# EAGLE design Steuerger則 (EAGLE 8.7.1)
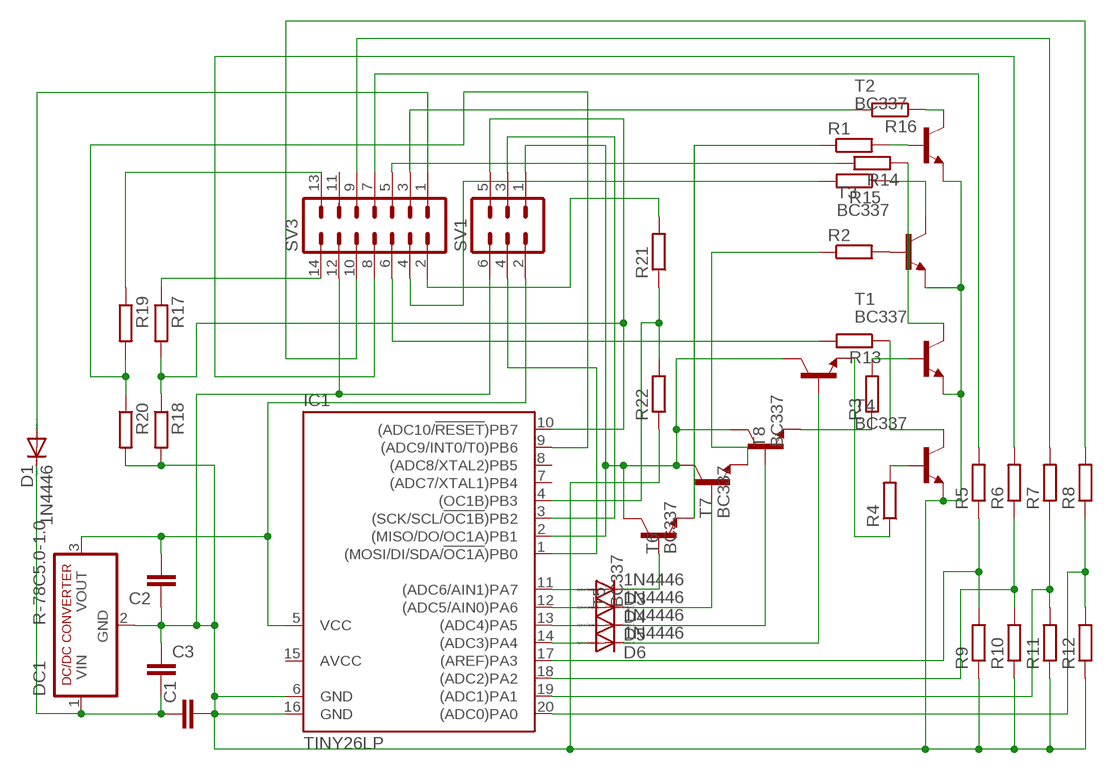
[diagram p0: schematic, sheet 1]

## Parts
C1  C5/3  [C5B3]
C2  C5/3  [C5B3]
C3  C5/3  [C5B3]
D1  1N4446  [DO35-10]
D3  1N4446  [DO35-10]
D4  1N4446  [DO35-10]
D5  1N4446  [DO35-10]
D6  1N4446  [DO35-10]
DC1  R-78C5.0-1.0  [SIP3]
IC1  TINY26LP  [DIL20]
R1  R-EU_0204/5  [0204/5]
R2  R-EU_0204/5  [0204/5]
R3  R-EU_0204/5  [0204/5]
R4  R-EU_0204/5  [0204/5]
R5  R-EU_0204/5  [0204/5]
R6  R-EU_0204/5  [0204/5]
R7  R-EU_0204/5  [0204/5]
R8  R-EU_0204/5  [0204/5]
R9  R-EU_0204/5  [0204/5]
R10  R-EU_0204/5  [0204/5]
R11  R-EU_0204/5  [0204/5]
R12  R-EU_0204/5  [0204/5]
R13  R-EU_0204/5  [0204/5]
R14  R-EU_0204/5  [0204/5]
R15  R-EU_0204/5  [0204/5]
R16  R-EU_0204/5  [0204/5]
R17  R-EU_0204/5  [0204/5]
R18  R-EU_0204/5  [0204/5]
R19  R-EU_0204/5  [0204/5]
R20  R-EU_0204/5  [0204/5]
R21  R-EU_0204/5  [0204/5]
R22  R-EU_0204/5  [0204/5]
SV1  ML6L  [ML6L]
SV3  ML14L  [ML14L]
T1  BC337  [TO92]
T2  BC337  [TO92]
T3  BC337  [TO92]
T4  BC337  [TO92]
T5  BC337  [TO92]
T6  BC337  [TO92]
T7  BC337  [TO92]
T8  BC337  [TO92]

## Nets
N$1: D1.A SV3.1
N$2: C2.2 DC1.3(VOUT) IC1.5(VCC) SV1.2
N$3: R17.1 SV3.14
N$4: IC1.3((SCK/SCL/!OC1B!)PB2) SV1.3
N$5: R19.1 SV3.13
N$6: IC1.1((MOSI/DI/SDA/!OC1A!)PB0) SV1.4
N$8: C1.2 C2.1 C3.1 DC1.2(GND) IC1.6(GND) IC1.16(GND) R9.1 R10.1 R11.1 R12.1 R18.2 R20.2 R22.1 SV1.6 SV3.12 T1.1(E) T2.1(E) T3.1(E) T4.1(E)
N$9: IC1.17((AREF)PA3) R5.1 R9.2
N$10: IC1.18((ADC2)PA2) R6.1 R10.2
N$11: IC1.19((ADC1)PA1) R7.1 R11.2
N$12: IC1.20((ADC0)PA0) R8.1 R12.2
N$14: D3.A IC1.11((ADC6/AIN1)PA7)
N$15: D4.A IC1.12((ADC5/AIN0)PA6)
N$16: D5.A IC1.13((ADC4)PA5)
N$17: D3.C T5.2(B)
N$18: D4.C T6.2(B)
N$19: D6.A IC1.14((ADC3)PA4)
N$20: R1.2 T2.2(B)
N$21: R2.2 T3.2(B)
N$22: R3.2 T1.2(B)
N$23: R4.2 T4.2(B)
N$24: D5.C T7.2(B)
N$25: D6.C T8.2(B)
N$26: R1.1 T5.1(E)
N$27: R2.1 T6.1(E)
N$28: R16.2 SV3.3
N$29: R15.2 SV3.4
N$30: R14.2 SV3.5
N$31: R13.2 SV3.6
N$32: R16.1 T2.3(C)
N$33: R13.1 T4.3(C)
N$34: R5.2 SV3.7
N$35: R6.2 SV3.8
N$36: R7.2 SV3.9
N$37: R8.2 SV3.10
N$38: R14.1 T1.3(C)
N$39: R15.1 T3.3(C)
N$40: R3.1 T7.1(E)
N$41: R4.1 T8.1(E)
N$42: IC1.9((ADC9/INT0/T0)PB6) R19.2 R20.1
N$43: C1.1 C3.2 D1.C DC1.1(VIN)
N$44: IC1.2((MISO/DO/OC1A)PB1) SV1.1 T5.3(C) T6.3(C) T7.3(C) T8.3(C)
N$45: IC1.10((ADC10/!RESET!)PB7) R17.2 R18.1 SV1.5
N$46: IC1.4((OC1B)PB3) R21.1 R22.2
N$47: R21.2 SV3.2
Unconnected: IC1.7((ADC7/XTAL1)PB4) IC1.8((ADC8/XTAL2)PB5) SV3.11

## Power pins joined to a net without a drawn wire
AVCC: IC1.15(AVCC)

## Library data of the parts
C1-C3 = capacitor-wima:C: CAPACITOR
D1 D3-D6 = diode:1N4446: DIODE
DC1 = dc-dc-converter:R-78C*-1.0: INNOLINE DC/DC-Converter 1.0 AMP SIP3 Single Output Source: Data sheet
IC1 = atmel:TINY26*: 8-bit AVR Microcontroller with 2K Bytes Flash Source: http://www.atmel.com .. doc1477.pdf; MPN: ATTINY26L-8PU; OC_FARNELL: 9171657; OC_NEWARK: 01M6920
R1-R4 R21 R22 = resistor:R-EU_: RESISTOR, European symbol
R5-R20 = rcl:R-EU_: RESISTOR, European symbol; SPICEPREFIX: R
SV1 = con-ml:ML6L: HARTING; OC_FARNELL: unknown; OC_NEWARK: unknown
SV3 = con-ml:ML14L: HARTING; OC_FARNELL: unknown; OC_NEWARK: unknown
T1-T8 = transistor:BC337: NPN TRANSISTOR

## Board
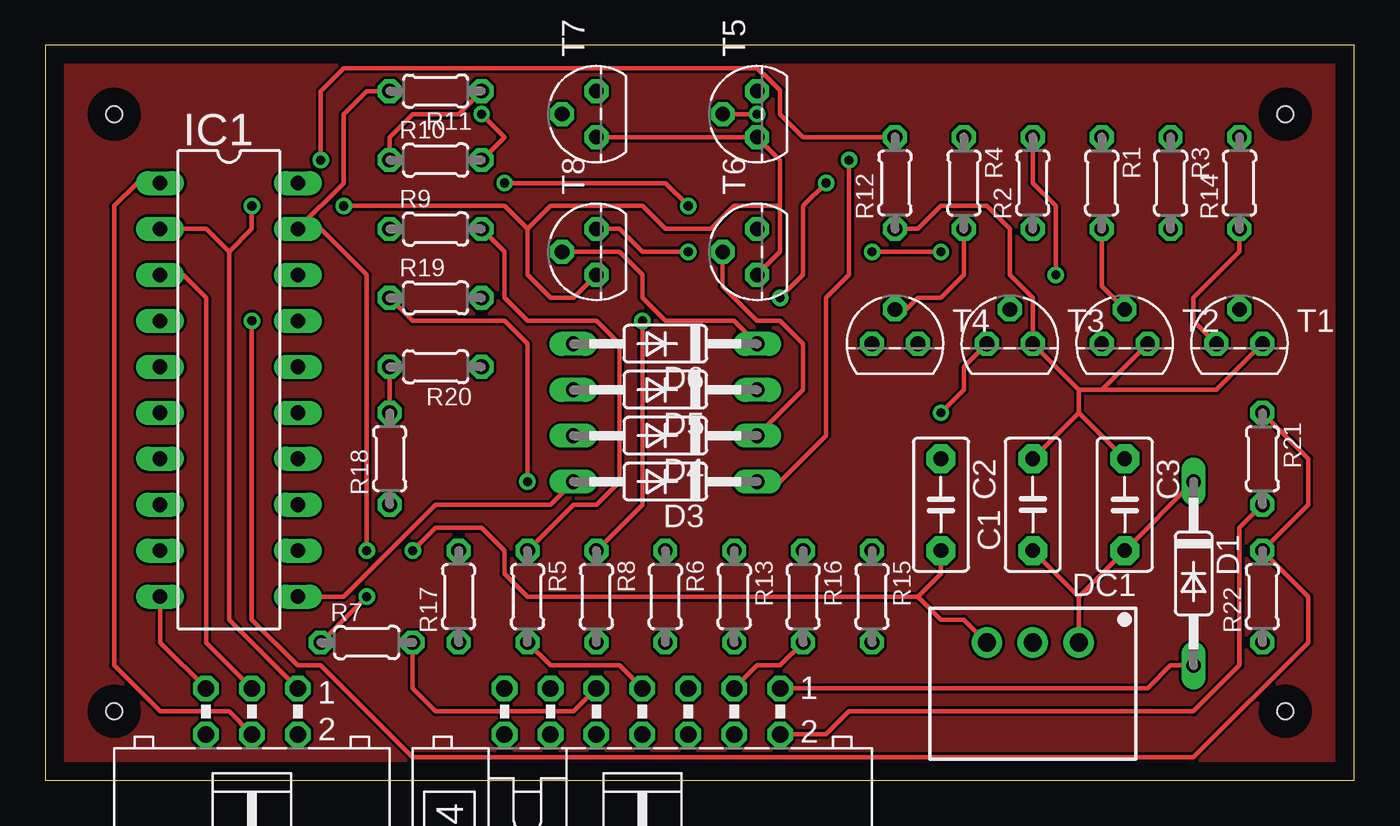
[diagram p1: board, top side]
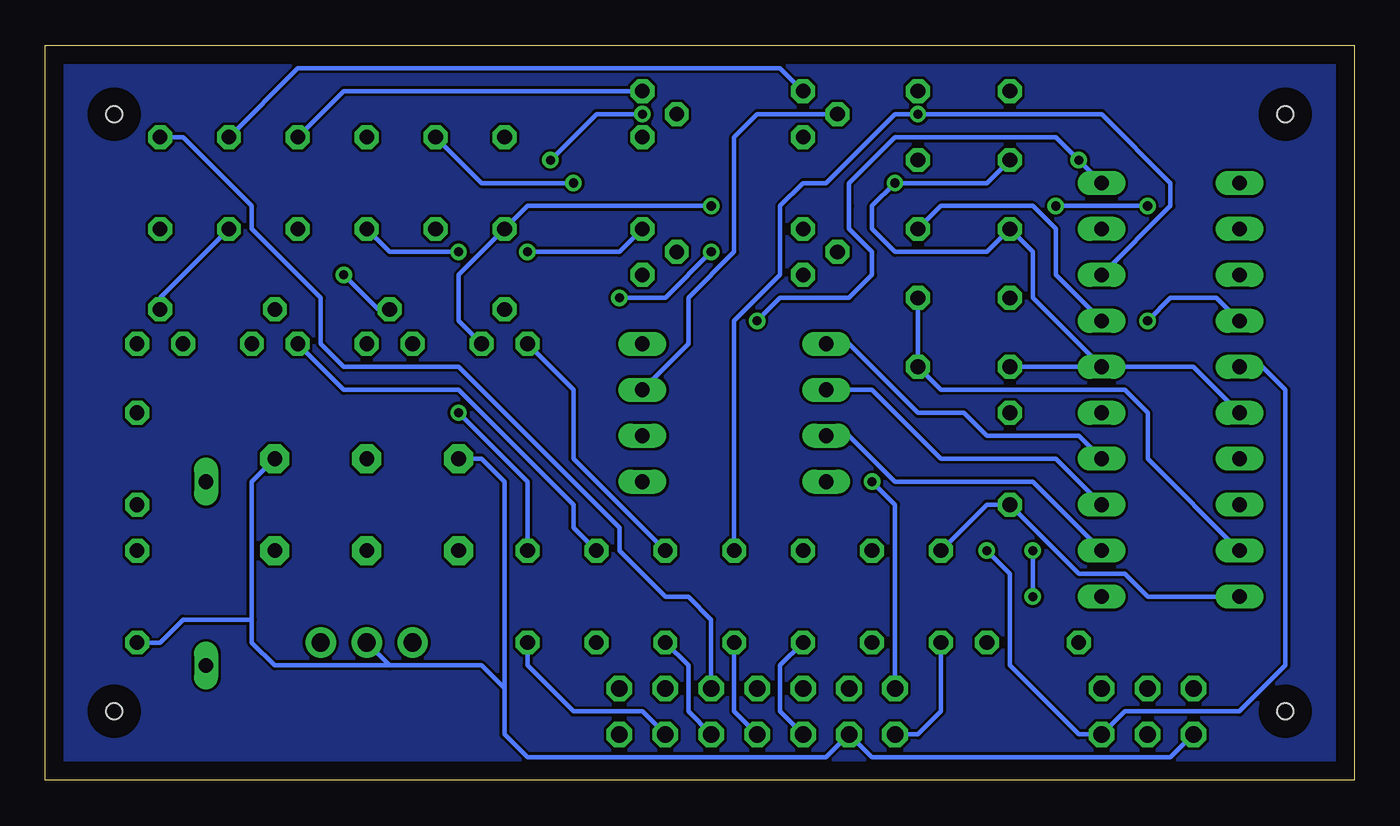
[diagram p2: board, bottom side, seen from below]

Size 72.39 x 40.64 mm. Coordinates in mm from the lower left corner, seen from the top.
Outline: 0,0 72.39,0 72.39,40.64 0,40.63 0,0
Copper layers (1*16): Top 0.035mm / dielectric 1.5mm / Bottom 0.035mm
Design rules "default": minimum track width 6mil, minimum drill 0.35mm, track to track 6mil, track to pad 6mil, pad to pad 6mil, via to via 6mil, smd to smd 6mil, copper to edge 40mil, drill to drill 6mil, minimum pad ring 10mil, minimum via ring 8mil, stop-mask expansion 4mil, vias tented up to drill 0mil, thermal gap 10mil
Holes 0.9 mm at 3.81,3.81 3.81,36.83 68.58,36.83 68.58,3.81

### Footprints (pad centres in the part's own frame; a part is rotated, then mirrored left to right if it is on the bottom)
C5B3 = drill 0.813 pad 1.6 octagon: 1 -2.54,0; 2 2.54,0
DO35-10 = drill 0.813 long: A 5.08,0; C -5.08,0
SIP3 = drill 1 pad 1.676: 1 -2.54,0; 2 0,0; 3 2.54,0
DIL20 = drill 0.813 long: 1 -11.43,-3.81; 2 -8.89,-3.81; 3 -6.35,-3.81; 4 -3.81,-3.81; 5 -1.27,-3.81; 6 1.27,-3.81; 7 3.81,-3.81; 8 6.35,-3.81; 9 8.89,-3.81; 10 11.43,-3.81; 11 11.43,3.81; 12 8.89,3.81; 13 6.35,3.81; 14 3.81,3.81; 15 1.27,3.81; 16 -1.27,3.81; 17 -3.81,3.81; 18 -6.35,3.81; 19 -8.89,3.81; 20 -11.43,3.81
0204/5 = drill 0.813 octagon: 1 -2.54,0; 2 2.54,0
ML6L = drill 0.914 octagon: 1 -2.54,-1.27; 2 -2.54,1.27; 3 0,-1.27; 4 0,1.27; 5 2.54,-1.27; 6 2.54,1.27
ML14L = drill 0.914 octagon: 1 -7.62,-1.27; 2 -7.62,1.27; 3 -5.08,-1.27; 4 -5.08,1.27; 5 -2.54,-1.27; 6 -2.54,1.27; 7 0,-1.27; 8 0,1.27; 9 2.54,-1.27; 10 2.54,1.27; 11 5.08,-1.27; 12 5.08,1.27; 13 7.62,-1.27; 14 7.62,1.27
TO92 = drill 0.813 octagon: 1 1.27,0; 2 0,1.905; 3 -1.27,0

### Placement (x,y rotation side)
C1  54.61,15.24 90 top
C2  49.53,15.24 270 top
C3  59.69,15.24 270 top
D1  63.5,11.43 270 top
D3  34.29,16.51 180 top
D4  34.29,19.05 180 top
D5  34.29,21.59 180 top
D6  34.29,24.13 180 top
DC1  54.61,7.62 180 top
IC1  10.16,21.59 270 top
R1  58.42,33.02 270 top
R2  54.61,33.02 90 top
R3  62.23,33.02 270 top
R4  50.8,33.02 270 top
R5  26.67,10.16 270 top
R6  34.29,10.16 270 top
R7  17.78,7.62 0 top
R8  30.48,10.16 270 top
R9  21.59,30.48 0 top
R10  21.59,34.29 0 top
R11  21.59,38.1 180 top
R12  46.99,33.02 90 top
R13  38.1,10.16 270 top
R14  66.04,33.02 90 top
R15  45.72,10.16 270 top
R16  41.91,10.16 270 top
R17  22.86,10.16 90 top
R18  19.05,17.78 90 top
R19  21.59,26.67 0 top
R20  21.59,22.86 180 top
R21  67.31,17.78 270 top
R22  67.31,10.16 90 top
SV1  11.43,3.81 180 top
SV3  33.02,3.81 180 top
T1  66.04,24.13 0 top
T2  59.69,24.13 0 top
T3  53.34,24.13 0 top
T4  46.99,24.13 0 top
T5  39.37,36.83 90 top
T6  39.37,29.21 90 top
T7  30.48,36.83 90 top
T8  30.48,29.21 90 top

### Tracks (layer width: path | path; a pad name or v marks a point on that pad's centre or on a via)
BOTTOM
  pour Bottom: 0,40.64 72.39,40.64 72.39,0 0,0
N$1
  Top 0.254: SV3.1 60.96,5.08 62.23,6.35 D1.A
N$2  (via drill 0.5)
  Top 0.254: v20.32,12.7 21.59,13.97 24.13,13.97 25.4,12.7 25.4,11.43 26.67,10.16 48.26,10.16 | 48.26,10.16 49.53,11.43 C2.2 | 48.26,10.16 49.53,8.89 50.8,8.89 DC1.3
  Bottom 0.254: IC1.5 5.08,22.86 3.81,21.59 3.81,6.35 6.35,3.81 12.7,3.81 SV1.2 15.24,2.54 19.05,6.35 19.05,11.43 v20.32,12.7
N$3
  Bottom 0.254: R17.1 22.86,3.81 24.13,2.54 SV3.14
N$4
  Top 0.254: IC1.3 7.62,27.94 8.89,26.67 8.89,7.62 SV1.3
N$5  (via drill 0.5)
  Top 0.254: v26.67,16.51 26.67,24.13 25.4,25.4 20.32,25.4 R19.1
  Bottom 0.254: SV3.13 25.4,15.24 v26.67,16.51
N$6
  Top 0.254: IC1.1 5.08,33.02 3.81,31.75 3.81,6.35 6.35,3.81 10.16,3.81 SV1.4
N$8  (via drill 0.5)
  Top 0.254: R20.2 R18.2 | R10.1 19.05,35.56 20.32,36.83 22.86,36.83 R11.1 | v35.56,31.75 34.29,33.02 v25.4,33.02 | R12.1 48.26,30.48 49.53,31.75 52.07,31.75 53.34,30.48 53.34,27.94 54.61,26.67 T3.1 57.15,21.59 | 57.15,21.59 58.42,21.59 | 58.42,21.59 T2.1 | 58.42,21.59 64.77,21.59 T1.1 | 57.15,21.59 57.15,20.32 | 57.15,20.32 C1.2 | C3.1 57.15,20.32
  Bottom 0.254: SV1.6 10.16,1.27 26.67,1.27 SV3.12 29.21,1.27 45.72,1.27 46.99,2.54 46.99,5.08 | 46.99,5.08 46.99,16.51 48.26,17.78 C2.1 | 46.99,5.08 48.26,6.35 53.34,6.35 | 53.34,6.35 DC1.2 | 53.34,6.35 59.69,6.35 60.96,7.62 60.96,8.89 | 60.96,8.89 60.96,16.51 C3.1 | IC1.6 8.89,22.86 IC1.16 | IC1.16 R20.2 | IC1.16 17.78,26.67 17.78,29.21 R9.1 20.32,29.21 25.4,29.21 26.67,30.48 26.67,31.75 v25.4,33.02 20.32,33.02 R10.1 | T4.1 49.53,25.4 49.53,27.94 R12.1 45.72,31.75 v35.56,31.75 | R22.1 66.04,7.62 64.77,8.89 60.96,8.89
N$9
  Top 0.254: R5.1 29.21,15.24 30.48,15.24 31.75,16.51 31.75,24.13 30.48,25.4 26.67,25.4 25.4,26.67 25.4,29.21 R9.2
  Bottom 0.254: IC1.17 16.51,27.94 16.51,30.48 17.78,31.75 22.86,31.75 R9.2
N$10  (via drill 0.5)
  Top 0.254: R10.2 25.4,35.56 v24.13,36.83
  Bottom 0.254: IC1.18 10.16,31.75 10.16,33.02 13.97,36.83 v24.13,36.83 25.4,36.83 29.21,33.02 30.48,33.02 31.75,31.75 31.75,27.94 34.29,25.4 R6.1
N$11  (via drill 0.5)
  Top 0.254: R11.2 17.78,38.1 16.51,36.83 16.51,33.02 IC1.19 15.24,30.48 17.78,27.94 v17.78,12.7 | R7.1 v17.78,10.16
  Bottom 0.254: v17.78,10.16 v17.78,12.7
N$12  (via drill 0.5)
  Top 0.254: R8.1 33.02,15.24 v33.02,25.4 | R12.2 41.91,35.56 40.64,36.83 40.64,38.16 39.76,39.04 39.7,39.04 39.37,39.37 16.51,39.37 15.24,38.1 v15.24,34.29
  Bottom 0.254: v33.02,25.4 31.75,26.67 27.94,26.67 26.67,27.94 26.67,29.21 27.94,30.48 27.94,31.75 27.94,33.02 25.4,35.56 16.51,35.56 v15.24,34.29 IC1.20
N$14
  Top 0.254: IC1.11 16.51,10.16 21.59,15.24 27.94,15.24 D3.A
N$15
  Bottom 0.254: IC1.12 17.78,16.51 25.4,16.51 27.94,19.05 D4.A
N$16
  Bottom 0.254: IC1.13 16.51,17.78 22.86,17.78 26.67,21.59 D5.A
N$17  (via drill 0.5)
  Top 0.254: T5.2 v39.37,36.83 | v44.45,34.29 44.45,27.94 43.18,26.67 43.18,19.05 40.64,16.51 D3.C
  Bottom 0.254: v39.37,36.83 41.91,36.83 v44.45,34.29
N$18
  Top 0.254: T6.2 37.47,27.31 39.37,25.4 40.64,25.4 41.91,24.13 41.91,21.59 D4.C
N$19
  Bottom 0.254: IC1.14 15.24,19.05 20.32,19.05 21.59,20.32 24.13,20.32 27.94,24.13 D6.A
N$20
  Top 0.254: R1.2 58.42,27.31 T2.2
N$21  (via drill 0.5)
  Top 0.254: R2.2 54.61,33.02 55.88,31.75 v55.88,27.94
  Bottom 0.254: v55.88,27.94 53.98,26.04 T3.2
N$22
  Bottom 0.254: R3.2 66.04,26.67 T1.2
N$23
  Top 0.254: T4.2 47.62,26.04 48.26,26.67 49.53,26.67 50.8,27.94 R4.2
N$24
  Bottom 0.254: T7.2 33.02,36.83 34.29,35.56 34.29,29.21 36.83,26.67 36.83,24.13 D5.C
N$25
  Top 0.254: D6.C 38.1,25.4 34.29,25.4 33.02,26.67 33.02,27.94 31.75,29.21 T8.2
N$26
  Bottom 0.254: T5.1 55.88,38.1 R1.1
N$27  (via drill 0.5)
  Top 0.254: v49.53,29.21 v45.72,29.21
  Bottom 0.254: R2.1 53.34,29.21 v49.53,29.21 | v45.72,29.21 40.64,29.21 T6.1
N$28
  Top 0.254: R16.2 40.64,6.35 39.37,6.35 SV3.3
N$29
  Bottom 0.254: R15.2 45.72,6.35 43.18,3.81 39.37,3.81 SV3.4
N$30
  Bottom 0.254: SV3.5 35.56,8.89 36.83,10.16 38.1,10.16 40.64,12.7 40.64,13.97 49.53,22.86 55.88,22.86 57.15,24.13 57.15,26.67 60.96,30.48 60.96,31.75 64.77,35.56 R14.2
N$31
  Bottom 0.254: R13.2 36.83,6.35 36.83,3.81 SV3.6
N$32
  Bottom 0.254: R16.1 43.18,13.97 43.18,15.24 49.53,21.59 55.88,21.59 T2.3
N$33
  Bottom 0.254: T4.3 43.18,21.59 43.18,17.78 R13.1
N$34
  Top 0.254: R5.2 27.94,6.35 31.75,6.35 SV3.7
N$35
  Bottom 0.254: R6.2 34.29,3.81 SV3.8
N$36
  Top 0.254: SV3.9 29.21,3.81 21.59,3.81 20.32,5.08 R7.2
N$37
  Bottom 0.254: SV3.10 31.75,3.81 31.75,6.35 R8.2
N$38
  Top 0.254: R14.1 66.04,29.21 63.5,26.67 63.5,25.4 T1.3
N$39  (via drill 0.5)
  Top 0.254: v49.53,20.32 50.8,21.59 50.8,22.86 T3.3
  Bottom 0.254: R15.1 45.72,16.51 v49.53,20.32
N$40
  Bottom 0.254: T7.1 31.75,39.37 58.42,39.37 R3.1
N$41  (via drill 0.5)
  Top 0.254: v43.18,33.02 41.91,31.75 41.91,27.94 v40.64,26.67 | v35.56,29.21 33.02,29.21 31.75,30.48 T8.1
  Bottom 0.254: R4.1 48.26,33.02 v43.18,33.02 | v40.64,26.67 38.1,26.67 v35.56,29.21
N$42
  Bottom 0.254: R19.2 R20.1 22.86,21.59 12.7,21.59 11.43,20.32 11.43,17.78 IC1.9
N$43
  Top 0.254: DC1.1 57.15,10.16 | 57.15,10.16 C1.1 | 57.15,10.16 C3.2 D1.C
N$44  (via drill 0.5)
  Top 0.254: IC1.2 8.89,30.48 10.16,29.21 | 10.16,29.21 10.16,8.89 SV1.1 | 10.16,29.21 11.43,30.48 v11.43,31.75 | v16.51,31.75 25.4,31.75 26.67,30.48 | 26.67,30.48 26.67,27.94 27.94,26.67 29.21,26.67 T8.3 | 26.67,30.48 27.94,31.75 33.02,31.75 34.29,30.48 36.83,30.48 38.1,31.75 40.64,31.75 | 40.64,31.75 40.64,34.29 T5.3 T7.3 | 40.64,31.75 40.64,29.21 T6.3
  Bottom 0.254: v11.43,31.75 v16.51,31.75
N$45
  Top 0.254: IC1.10 6.35,7.62 SV1.5
  Bottom 0.254: IC1.10 11.43,10.16 12.7,11.43 15.24,11.43 R18.1 20.32,15.24 R17.2
N$46  (via drill 0.5)
  Top 0.254: v11.43,25.4 11.43,8.89 13.97,6.35 15.24,6.35 20.32,1.27 63.5,1.27 69.85,7.62 69.85,10.16 R22.2 69.85,15.24 69.85,17.78 R21.1
  Bottom 0.254: v11.43,25.4 10.16,26.67 7.62,26.67 IC1.4
N$47
  Top 0.254: R21.2 66.04,13.97 66.04,6.35 63.5,3.81 44.45,3.81 43.18,2.54 SV3.2
TOP
  pour Top: 0,40.64 72.39,40.64 72.39,0 0,0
